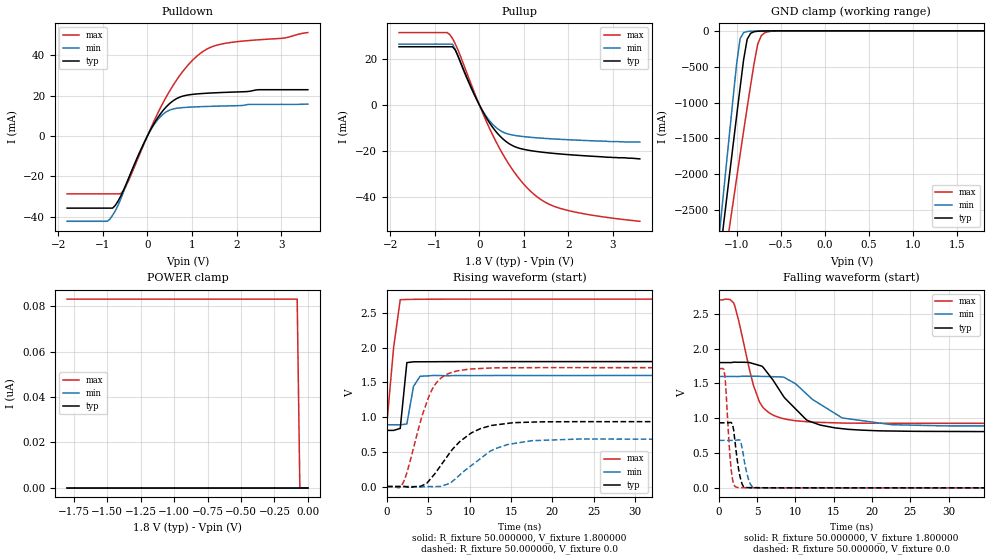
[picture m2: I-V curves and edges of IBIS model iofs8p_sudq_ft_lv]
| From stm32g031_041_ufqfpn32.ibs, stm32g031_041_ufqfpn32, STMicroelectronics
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|   Model iofs8p_sudq_ft_lv
[Model]  iofs8p_sudq_ft_lv
Model_type I/O
Polarity   Non-Inverting
Enable   Active-Low
Vinl =   0.540000V
Vinh =   1.260000V
Vmeas =  0.900000V
Cref =   40.000000pF
Rref =   100.000000M
Vref =   0.0V
C_comp   1.984800pF   1.899400pF   2.077500pF
[Temperature Range]   25.000000   -40.000000   0.125000k
[Pullup Reference]   1.800000V   1.600000V   2.700000V
[Pulldown Reference]   0.0V   0.0V   0.0V
[POWER Clamp Reference]   1.800000V   1.600000V   2.700000V
[GND Clamp Reference]   0.0V   0.0V   0.0V
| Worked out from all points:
|   slope of the pulldown table from 0 to 0.27 V, typ, clamps not added: 26.4 ohm
|   slope of the pullup table from 0 to 0.27 V, typ, clamps not added: 30.1 ohm
|   GND clamp passes 1 mA (typ) near -0.61 V on its own axis
|   rising waveform, R_fixture 50.000000, V_fixture 1.800000: 20-80 % time 502ps typ, 696ps min, 936ps max; typ from 0.809 V to 1.8 V
|   rising waveform, R_fixture 50.000000, V_fixture 0.0: 20-80 % time 4.11ns typ, 4.63ns min, 2.6ns max; typ from 0 V to 0.934 V
|   falling waveform, R_fixture 50.000000, V_fixture 1.800000: 20-80 % time 4.46ns typ, 5.33ns min, 2.44ns max; typ from 1.8 V to 0.809 V
|   falling waveform, R_fixture 50.000000, V_fixture 0.0: 20-80 % time 695ps typ, 761ps min, 597ps max; typ from 0.934 V to 0 V
[Pulldown]
|Voltage   I(typ)   I(min)   I(max)
-1.8V     -35.64mA   -42.15mA   -28.59mA
-900mV    -35.64mA   -42.15mA   -28.59mA
-780mV    -35.64mA   -39.2mA    -28.59mA
-600mV    -29.83mA   -31.3mA    -28.52mA
-420mV    -20.8mA    -21.07mA   -21.98mA
60mV      2.604mA    2.459mA    3.062mA
240mV     9.303mA    8.31mA     11.61mA
480mV     15.67mA    12.64mA    21.52mA
720mV     19.18mA    13.9mA     29.74mA
960mV     20.46mA    14.3mA     36.27mA
1.44V     21.29mA    14.7mA     44.06mA
3.6V      22.91mA    15.79mA    51.15mA
[Pullup]
|Voltage   I(typ)   I(min)   I(max)
-1.8V     25.2mA     26.35mA    31.36mA
-660mV    25.2mA     26.35mA    30.47mA
-600mV    25.2mA     26.35mA    28.77mA
-540mV    23.79mA    24.11mA    26.53mA
-60mV     2.392mA    2.26mA     2.893mA
300mV     -9.801mA   -8.48mA    -13.12mA
480mV     -13.91mA   -11.33mA   -19.82mA
720mV     -17.48mA   -13.04mA   -27.46mA
1.26V     -20.22mA   -14.3mA    -39.41mA
1.56V     -20.9mA    -14.71mA   -43.14mA
1.98V     -21.62mA   -15.16mA   -45.85mA
3.6V      -23.5mA    -16.2mA    -50.6mA
[GND_clamp]
|Voltage   I(typ)   I(min)   I(max)
-1.8V     -9.477A    -9.805A    -9.016A
-1.2V     -3.243A    -2.9A      -3.759A
-1.16V    -2.83A     -2.409A    -3.417A
-1.12V    -2.418A    -1.919A    -3.076A
-1.08V    -2.008A    -1.431A    -2.736A
-1V       -1.194A    -466mA     -2.061A
-960mV    -792.8mA   -108.7mA   -1.727A
-920mV    -402mA     -24.35mA   -1.396A
-880mV    -117.8mA   -9.188mA   -1.071A
-760mV    -5.896mA   -2.88mA    -183.8mA
-680mV    -2.395mA   -1.099mA   -26.61mA
1.8V      0A         0A         0A
[POWER_clamp]
|Voltage   I(typ)   I(min)   I(max)
-1.8V     0A         0A         83.17nA
-80mV     0A         0A         83.17nA
-60mV     0A         0A         0A
0V        0A         0A         0A
[Ramp]
| variable   typ   min   max
dV/dt_r  0.56056/4.10615n   0.40980/4.64093n   1.02750/2.59632n
dV/dt_f  0.59503/4.45986n   0.42595/5.32206n   1.06403/2.43879n
R_load = 50.000000
[Rising Waveform]
R_fixture= 50.000000
V_fixture= 1.800000
V_fixture_min= 1.600000
V_fixture_max= 2.700000
|time   V(typ)   V(min)   V(max)
0s        808.8mV    889.5mV    927.1mV
800.8ps   808.5mV    889.6mV    2.002V
1.602ns   837.1mV    889.6mV    2.691V
2.402ns   1.785V     900.6mV    2.695V
3.203ns   1.797V     1.441V     2.697V
4.004ns   1.798V     1.589V     2.698V
5.606ns   1.798V     1.6V       2.699V
79.28ns   1.8V       1.6V       2.7V
[Rising Waveform]
R_fixture= 50.000000
V_fixture= 0.0
V_fixture_min= 0.0
V_fixture_max= 0.0
|time   V(typ)   V(min)   V(max)
0s        959.8nV    708.2nV    1.585uV
1.441ns   16.71uV    -614.4nV   -19.31mV
2.082ns   -221.6uV   113.9nV    88.06mV
4.324ns   17.14mV    -4.672mV   1.047V
5.766ns   180.8mV    -549.2uV   1.46V
6.887ns   367.2mV    16.92mV    1.593V
8.649ns   628.5mV    150.9mV    1.669V
12.49ns   874.9mV    510.7mV    1.707V
17.62ns   928.3mV    661.2mV    1.712V
79.76ns   934.4mV    682.2mV    1.713V
[Falling Waveform]
R_fixture= 50.000000
V_fixture= 1.800000
V_fixture_min= 1.600000
V_fixture_max= 2.700000
|time   V(typ)   V(min)   V(max)
0s        1.8V       1.6V       2.7V
1.922ns   1.806V     1.6V       2.659V
4.484ns   1.784V     1.604V     1.483V
5.285ns   1.759V     1.603V     1.238V
8.809ns   1.268V     1.57V      985.4mV
11.53ns   969.6mV    1.341V     949.9mV
13.13ns   905.6mV    1.208V     940.8mV
16.18ns   849.5mV    1.003V     931.2mV
22.58ns   816.6mV    907.5mV    927.8mV
79.76ns   808.8mV    889.5mV    927.1mV
[Falling Waveform]
R_fixture= 50.000000
V_fixture= 0.0
V_fixture_min= 0.0
V_fixture_max= 0.0
|time   V(typ)   V(min)   V(max)
0s        934.4mV    682.2mV    1.713V
800.8ps   934.4mV    682.2mV    1.597V
1.602ns   938.8mV    682.1mV    262.9mV
1.922ns   834.4mV    681.7mV    54.04mV
2.402ns   394.4mV    687.1mV    6.141mV
2.883ns   107.8mV    648.8mV    3.044mV
3.203ns   19.14mV    464mV      2.445mV
4.004ns   2.658mV    80.78mV    1.546mV
4.645ns   1.907mV    3.998mV    1.127mV
79.76ns   959.8nV    708.2nV    1.585uV
